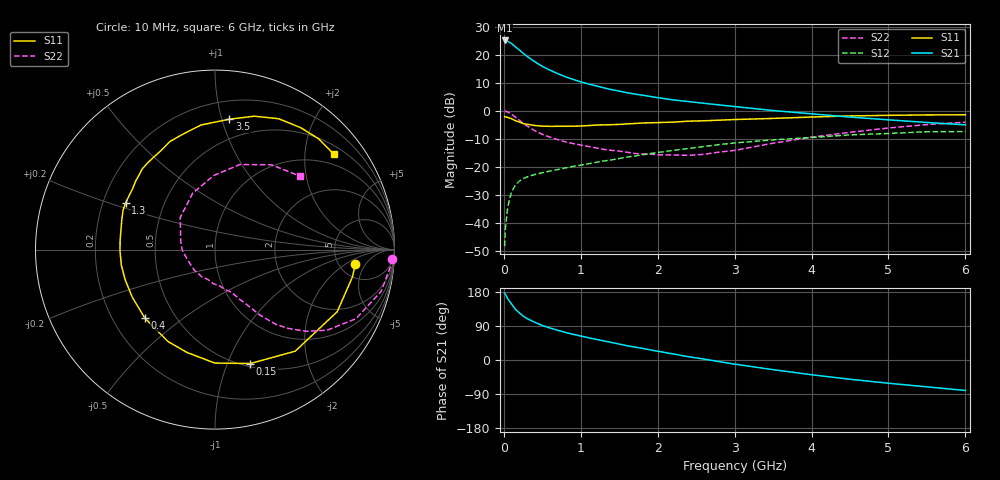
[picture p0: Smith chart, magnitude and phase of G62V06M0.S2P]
! SIEMENS Small Signal Semiconductors
! BFG193
! Si NPN RF Bipolar Junction Transistor in SOT223
! VCE = 2 V  IC = 6 mA
! Common Emitter S-Parameters:  August  1996
# GHz  S  MA  R  50
!  f  S11  S21  S12  S22
! GHz  MAG  ANG  MAG  ANG  MAG  ANG  MAG  ANG
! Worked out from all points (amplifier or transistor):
!   36 points, 10 MHz to 6 GHz, reference 50 ohm
!   highest |S21| = 25.2 dB at 10 MHz (marker M1)
!   |S21| within 3 dB of that: start of sweep to 182.9 MHz
!   unconditionally stable (mu >= 1): 1.009 GHz to 2.694 GHz
!   at 250 MHz: K = 0.39, MSG = 22.4 dB, |S12| = -24.3 dB
!   at 1.4 GHz: K = 1.09, MAG = 10.7 dB, |S12| = -17.5 dB
!   at 6 GHz: K = 0.91, MSG = 1.2 dB, |S12| = -7.4 dB
!   S11 on the Smith chart (normalised r, x): 10 MHz: 7.14, -2.92; 150 MHz: 0.53, -1.21; 400 MHz: 0.34, -0.37; 1.3 GHz: 0.30, +0.23; 3.5 GHz: 0.34, +1.06; 6 GHz: 0.70, +2.68
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0.01  0.7862 -5.7  18.12 176.2  0.0038 91.0  0.9887 -2.9
0.02  0.7809 -11.2  18.08 173.5  0.0076 85.0  0.9809 -5.8
0.05  0.7639 -26.9  17.52 161.8  0.0191 77.2  0.9548 -14.1
0.1  0.7212 -51.7  15.96 147.8  0.0356 66.7  0.8749 -26.1
0.15  0.6645 -72.8  13.95 133.9  0.0469 56.5  0.7694 -35.7
0.2  0.6321 -90.1  12.28 124.6  0.0551 51.7  0.6833 -41.8
0.25  0.5939 -105.2  10.74 116.1  0.0613 47.0  0.5994 -47.1
0.3  0.5754 -117.0  9.481 109.6  0.0657 44.5  0.5381 -50.8
0.4  0.5464 -135.7  7.577 99.7  0.0725 41.4  0.4435 -55.5
0.5  0.5318 -150.0  6.229 91.1  0.0781 39.4  0.3796 -58.4
0.6  0.528 -161.1  5.331 84.4  0.084 39.5  0.3384 -61.1
0.7  0.529 -170.5  4.633 78.4  0.0892 39.2  0.3061 -63.9
0.9  0.5311 174.5  3.646 67.8  0.1016 39.4  0.2593 -68.3
1.1  0.5445 162.5  3.019 58.8  0.1132 39.6  0.2307 -75.4
1.3  0.5614 152.4  2.581 50.3  0.127 38.9  0.2044 -82.4
1.6  0.5839 139.2  2.106 37.7  0.1484 36.8  0.182 -97.2
2.2  0.6283 118.6  1.569 16.0  0.1961 29.5  0.1624 -134.9
2.8  0.68 101.3  1.273 -4.3  0.2489 19.2  0.1828 -179.5
3.5  0.7311 83.7  1.012 -25.5  0.3023 3.7  0.2638 137.3
4.5  0.8107 64.1  0.773 -50.8  0.3709 -16.2  0.4128 91.0
5.5  0.8452 46.9  0.619 -70.9  0.4223 -40.8  0.567 56.5
6  0.8489 38.8  0.561 -80.4  0.4268 -54.7  0.6263 40.8
